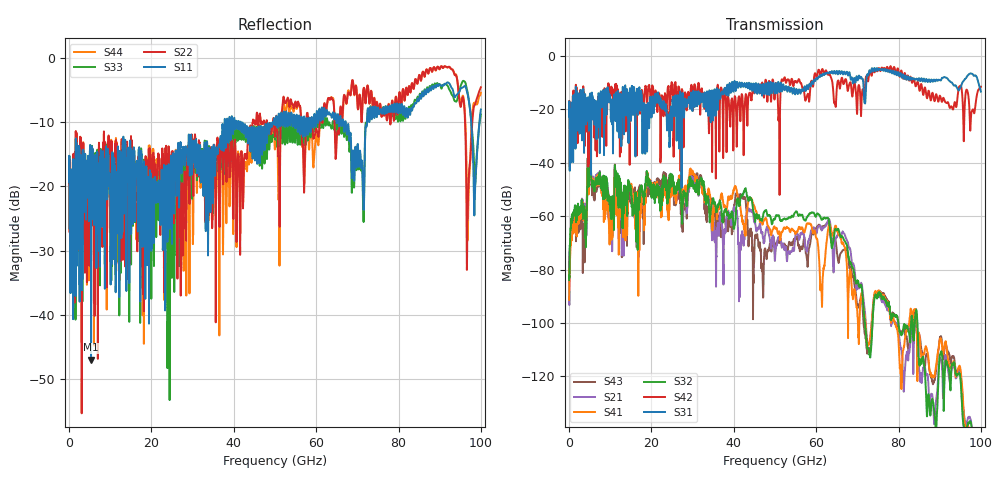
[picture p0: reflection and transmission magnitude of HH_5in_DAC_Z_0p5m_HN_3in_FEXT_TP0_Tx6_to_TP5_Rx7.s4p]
# GHz S RI R 45
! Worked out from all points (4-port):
!   4000 points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, 25 MHz to 100 GHz, reference 45 ohm
!   strongest paths, dB at 25 MHz, 25.02 GHz, 50.02 GHz, 75.03 GHz, 100 GHz:
!     S31: -22.7, -27.8, -12.7, -5.4, -13.3
!     S42: -22.5, -11.1, -12.9, -5.1, -11.5
!     S32: -83.9, -44.4, -61.0, -90.1, -177.1
!     S41: -91.3, -47.0, -64.4, -89.1, -180.2
!     S21: -88.6, -46.0, -76.2, -90.0, -175.1
!     S43: -87.8, -45.1, -73.4, -89.4, -182.3
!   lowest |S11| = -47.0 dB at 5.35 GHz (marker M1), VSWR 1.01, Z = 44.8 - j0.354 ohm
!   |S11| at or under -10 dB: start of sweep to 37.76 GHz; 41.71 GHz to 49.4 GHz (7.688 GHz wide, 16.9 % of centre); 67.18 GHz to 72.34 GHz (5.159 GHz wide, 7.4 % of centre)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
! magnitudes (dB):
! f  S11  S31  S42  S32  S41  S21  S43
! 25 MHz  -19.2  -22.7  -22.5  -83.9  -91.3  -88.6  -87.8
! 5.35 GHz  -47.0  -44.5  -22.9  -44.6  -44.2  -43.6  -46.1
! 10.1 GHz  -35.3  -19.3  -13.9  -57.7  -63.1  -60.5  -56.7
! 29.77 GHz  -14.5  -14.4  -11.6  -48.7  -44.2  -47.0  -45.9
! 46.92 GHz  -14.4  -14.1  -10.0  -61.3  -62.9  -65.9  -78.8
! 96.9 GHz  -6.0  -7.1  -14.2  -137.3  -138.5  -135.3  -141.4
! 100 GHz  -8.0  -13.3  -11.5  -177.1  -180.2  -175.1  -182.3
